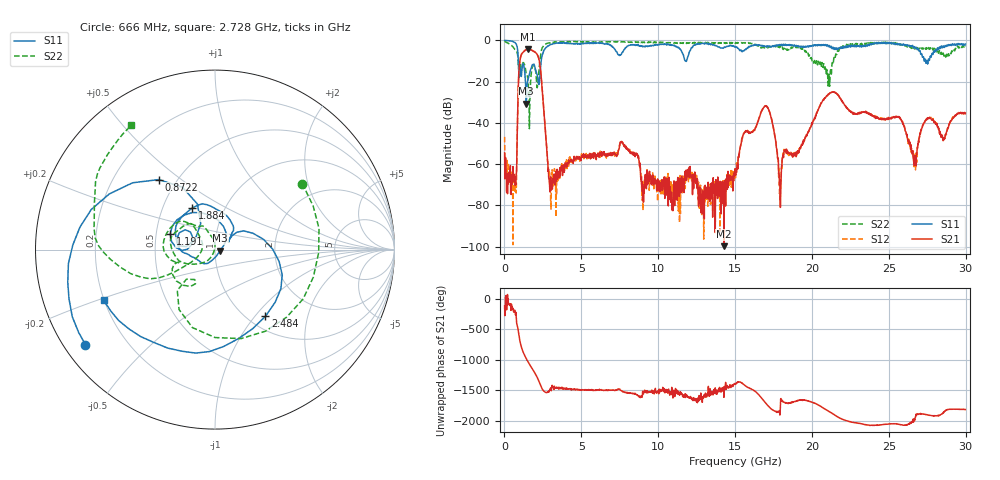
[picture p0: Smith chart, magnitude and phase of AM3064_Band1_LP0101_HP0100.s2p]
# Hz S DB R 50.0
!freq dBS11 angS11 dBS21 angS21 dBS12 angS12 dBS22 angS22
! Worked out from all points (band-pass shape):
!   1600 points, 10 MHz to 29.98 GHz, reference 50 ohm
!   highest |S21| = -4.27 dB at 1.528 GHz (marker M1); lowest = -99.8 dB at 14.27 GHz (marker M2)
!   |S21| within 3 dB of the highest: 1.08 GHz to 2.159 GHz (1.078 GHz wide, 66.6 % of centre)
!   lowest |S11| = -30.7 dB at 1.416 GHz (marker M3), VSWR 1.06, Z = 53 - j0.548 ohm
!   |S11| at or under -10 dB: 902 MHz to 2.389 GHz (1.486 GHz wide, 90.3 % of centre); 11.77 GHz to 11.84 GHz (66.96 MHz wide, 0.567 % of centre); 27.49058 GHz to 27.5639 GHz (73.32 MHz wide, 0.266 % of centre)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
!   |S22| runs from -42.8 to -0.4 dB; largest |S21 - S12| = 0.009
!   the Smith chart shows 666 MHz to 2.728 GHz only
!   S11 on the Smith chart (normalised r, x): 666 MHz: 0.06, -0.33; 872.2 MHz: 0.40, +0.42; 1.191 GHz: 0.59, +0.11; 1.884 GHz: 0.70, +0.35; 2.484 GHz: 1.20, -1.13; 2.728 GHz: 0.20, -0.21
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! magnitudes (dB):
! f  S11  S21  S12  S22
! 10 MHz  0.0  -54.6  -46.8  -0.4
! 666 MHz  -1.0  -66.0  -73.1  -4.3
! 872.2 MHz  -6.0  -30.8  -30.7  -8.2
! 1.191 GHz  -11.6  -5.9  -5.8  -10.9
! 1.416 GHz  -30.7  -4.5  -4.4  -16.1
! 1.528 GHz  -19.2  -4.3  -4.2  -19.6
! 1.884 GHz  -11.6  -5.2  -5.2  -11.9
! 2.484 GHz  -6.6  -26.3  -26.2  -3.3
! 2.728 GHz  -3.3  -50.2  -50.3  -1.6
! 3.084 GHz  -1.9  -68.3  -68.6  -1.1
! 5.015 GHz  -1.5  -56.5  -55.0  -0.7
! 7.657 GHz  -5.9  -49.6  -49.4  -0.7
! 10 GHz  -2.0  -69.6  -68.8  -0.9
! 14.27 GHz  -3.4  -99.8  -76.9  -1.4
! 15 GHz  -3.1  -62.2  -64.1  -1.4
! 16.92 GHz  -2.8  -32.0  -32.0  -3.6
! 17.91 GHz  -2.0  -67.7  -71.7  -3.3
! 19.99 GHz  -2.8  -40.7  -40.9  -9.4
! 21.32 GHz  -4.0  -25.0  -25.0  -10.7
! 25 GHz  -1.1  -37.6  -37.9  -1.2
! 26.66 GHz  -3.1  -60.8  -59.7  -4.0
! 29.98 GHz  -1.7  -35.3  -35.1  -2.8
